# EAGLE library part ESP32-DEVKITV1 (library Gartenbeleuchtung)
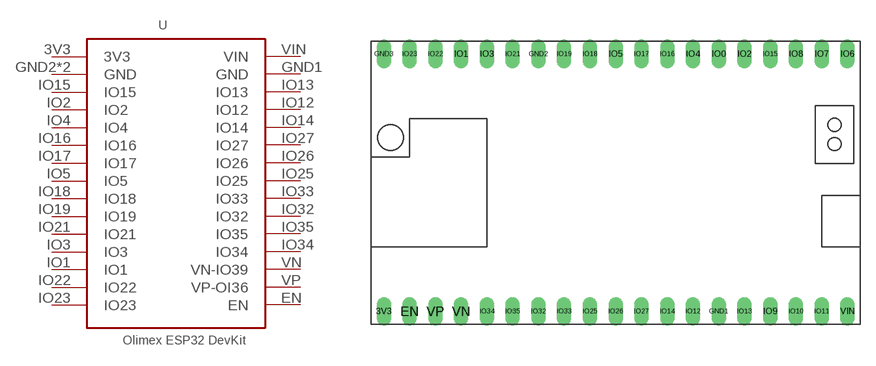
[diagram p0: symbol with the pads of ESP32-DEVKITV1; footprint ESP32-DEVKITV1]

Designator prefix -

## ESP32-DEVKITV1  [ESP32-DEVKITV1]
3V3  3V3  pwr
EN  EN
GND1  GND  pwr
GND2  GND  pwr
GND3  GND  pwr
IO1  IO1
IO2  IO2
IO3  IO3
IO4  IO4
IO5  IO5
IO12  IO12
IO13  IO13
IO14  IO14
IO15  IO15
IO16  IO16
IO17  IO17
IO18  IO18
IO19  IO19
IO21  IO21
IO22  IO22
IO23  IO23
IO25  IO25
IO26  IO26
IO27  IO27
IO32  IO32
IO33  IO33
IO34  IO34
IO35  IO35
VIN  VIN  pwr
VN  VN-IO39
VP  VP-OI36

## Footprint ESP32-DEVKITV1 (pad centres in mm)
drill 0.8 pad 1.422 long: 3V3 -22.86,-12.7; EN -20.32,-12.7; GND1 10.16,-12.7; GND2 -7.62,12.7; GND3 -22.86,12.7; IO0 10.16,12.7; IO1 -15.24,12.7; IO2 12.7,12.7; IO3 -12.7,12.7; IO4 7.62,12.7; IO5 0,12.7; IO6 22.86,12.7; IO7 20.32,12.7; IO8 17.78,12.7; IO9 15.24,-12.7; IO10 17.78,-12.7; IO11 20.32,-12.7; IO12 7.62,-12.7; IO13 12.7,-12.7; IO14 5.08,-12.7; IO15 15.24,12.7; IO16 5.08,12.7; IO17 2.54,12.7; IO18 -2.54,12.7; IO19 -5.08,12.7; IO21 -10.16,12.7; IO22 -17.78,12.7; IO23 -20.32,12.7; IO25 -2.54,-12.7; IO26 0,-12.7; IO27 2.54,-12.7; IO32 -7.62,-12.7; IO33 -5.08,-12.7; IO34 -12.7,-12.7; IO35 -10.16,-12.7; VIN 22.86,-12.7; VN -15.24,-12.7; VP -17.78,-12.7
